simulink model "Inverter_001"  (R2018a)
settings: Solver=FixedStepDiscrete  StartTime=0.0  StopTime=inf  RelTol=1e-3  EnableMultiTasking=on
PreLoadFcn:
  | Sample_Time
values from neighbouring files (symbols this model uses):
  C_filt = 9.2e-6    (= 9.2e-06)    [master5.m]    (also in Sample_Time.m = 1.175e-06)
  Kcp = 5 /2    (= 2.5)    [master5.m]    (also in Parametri_final.m = Kcp_rac*20; Sample_Time.m = 8.8)
  Kcp0 = 5 /2    (= 2.5)    [master5.m]    (also in Parametri_final.m = Kc0p_rac*20; Sample_Time.m = 8.8)
  Kvp = 1    [master5.m]    (also in Parametri_final.m = 0.06652; Sample_Time.m = 2.4)
  Kvp0 = 1    [master5.m]    (also in Parametri_final.m = 0.06652; Sample_Time.m = 2.4)
  L_filt = 1e-3    (= 0.001)    [master5.m]    (also in Sample_Time.m = 0.01)
  Tcontrol = 5e-5     *2    (= 0.0001)    [Sample_Time.m]
  Tmeasure = 5e-5    (= 5e-05)    [Sample_Time.m]
  w = 2*pi*50    (= 314.159265359)    [master5.m]    (also in Parametri_final.m = 314.1592)
undefined symbols (not defined in the file or in its folder): A, ADCIN0, ADCIN1, ADCINA0, ADCINB0, bit, C_filtEST, CC_Tci, CC_Tci0, CC_Tcr, Compare, Control, conversion, DCAEVT1, DCAEVT1FILT, Digital, Down, ended, Event, Filtered, GPTRIP1SEL, GPTRIP2SEL, input, Module, of, Single, start, Trip, TZ1, TZ2, Up, VC_Tci, VC_Tci0, VC_Tcr, version, Zone
libraries: tiiqmathlib x92, etargetslib x20, c2802xlib x13, c2837xDlib x7, c28xdmclib x1
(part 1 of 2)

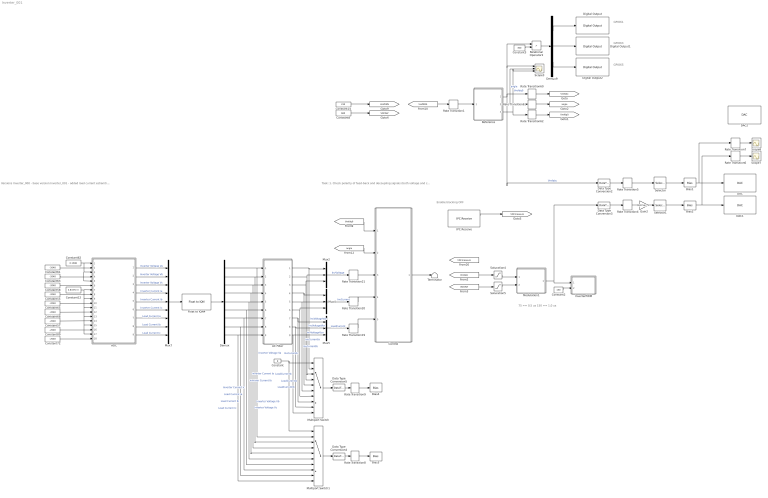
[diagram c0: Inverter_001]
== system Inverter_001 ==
  note: Enable blocking OFF
  note: Versions Inverter_000 - base version Inverter_001 - added load current estiamtion in control block
  note: Task: 1. Check polarity of feed-back and decoupling signals (both voltage and current control)
  note: 75 == 0,5 us 150 == 1,0 us
  note: GPIO61
  note: GPIO63
  note: GPIO65
  AC Filter : Subsystem
  ADC : Subsystem
  Bias1 : Bias  Bias=400
  Bias2 : Bias  Bias=400
  Bias3 : Bias  Commented=on  Bias=400
  Bias4 : Bias  Commented=on  Bias=400
  Constant : Constant  Commented=on  Value=9
  Constant12 : Constant  Value=4.8337e-3  OutDataTypeStr=single  SampleTime=0.1
  Constant14 : Constant  Value=230  OutDataTypeStr=single  SampleTime=Tcontrol
  Constant2 : Constant  Value=150  OutDataTypeStr=single
  Constant3 : Constant  Value=300  OutDataTypeStr=fixdt(1,32,2^-10,0)
  Constant{55,57..58,61,63,65,68,72,89} (9 alike) : Constant  Value=-2048  OutDataTypeStr=single  SampleTime=0.1
  Constant62 : Constant  Value=0.1588  OutDataTypeStr=single  SampleTime=0.1
  Constant8 : Constant  Value=680  OutDataTypeStr=fixdt(1,32,2^-10,0)
  Control : Subsystem
  DAC : c2837xDlib/DAC  channel=A  saturate=off
  DAC1 : c2837xDlib/DAC  channel=B  saturate=off
  DAC2 : c2837xDlib/DAC  channel=C  saturate=off
  Data Type Conversion2 : DataTypeConversion  OutDataTypeStr=single
  Data Type Conversion3 : DataTypeConversion  OutDataTypeStr=single
  Data Type Conversion4 : DataTypeConversion  Commented=on  OutDataTypeStr=single
  Data Type Conversion5 : DataTypeConversion  Commented=on  OutDataTypeStr=single
  Demux : Demux  Outputs=9
  Demux9 : Demux  Outputs=3
  Digital Output : c2837xDlib/Digital Output  GPIO_Number=GPIO56~GPIO63  GPIO_Bit0=off  GPIO_BIT0_Toggle=off  GPIO_Bit1=off  GPIO_BIT1_Toggle=off  GPIO_Bit2=off  GPIO_BIT2_Toggle=off  GPIO_Bit3=off  GPIO_BIT3_Toggle=off  GPIO_Bit4=off  GPIO_BIT4_Toggle=off  GPIO_Bit5=on  GPIO_BIT5_Toggle=off  GPIO_Bit6=off  GPIO_BIT6_Toggle=off  GPIO_Bit7=off  GPIO_BIT7_Toggle=off
  Digital Output1 : c2837xDlib/Digital Output  GPIO_Number=GPIO56~GPIO63  GPIO_Bit0=off  GPIO_BIT0_Toggle=off  GPIO_Bit1=off  GPIO_BIT1_Toggle=off  GPIO_Bit2=off  GPIO_BIT2_Toggle=off  GPIO_Bit3=off  GPIO_BIT3_Toggle=off  GPIO_Bit4=off  GPIO_BIT4_Toggle=off  GPIO_Bit5=off  GPIO_BIT5_Toggle=off  GPIO_Bit6=off  GPIO_BIT6_Toggle=off  GPIO_Bit7=on  GPIO_BIT7_Toggle=off
  Digital Output2 : c2837xDlib/Digital Output  GPIO_Number=GPIO64~GPIO71  GPIO_Bit0=off  GPIO_BIT0_Toggle=off  GPIO_Bit1=off  GPIO_BIT1_Toggle=off  GPIO_Bit2=on  GPIO_BIT2_Toggle=off  GPIO_Bit3=off  GPIO_BIT3_Toggle=off  GPIO_Bit4=off  GPIO_BIT4_Toggle=off  GPIO_Bit5=off  GPIO_BIT5_Toggle=off  GPIO_Bit6=off  GPIO_BIT6_Toggle=off  GPIO_Bit7=off  GPIO_BIT7_Toggle=off
  Float to IQN4 : tiiqmathlib/Float to IQN  Q_value=10
  Gain2 : Gain  Gain=230*sqrt(2)
  IPC Receive : c2837xDlib/IPC Receive  SelectChannel=0  DataType=single  DataLength=1  EnableBlocking=off  SampleTime=Tcontrol
  InverterPWM : Subsystem
  Modulation1 : Subsystem
  Multiport Switch : MultiPortSwitch  Commented=on  Inputs=9
  Multiport Switch1 : MultiPortSwitch  Commented=on  Inputs=9
  Mux2 : Mux  Inputs=3
  Mux4 : Mux  Inputs=3
  Mux5 : Mux  Inputs=3
  Mux7 : Mux  Inputs=9
  Rate Transition1 : RateTransition  OutPortSampleTime=5e-5
  Rate Transition{4..5,19..21,60..62} (8 alike) : RateTransition  OutPortSampleTime=Tcontrol
  Rate Transition6 : RateTransition  OutPortSampleTime=2e-4
  Rate Transition7 : RateTransition  OutPortSampleTime=2e-4
  Rate Transition8 : RateTransition  Commented=on  OutPortSampleTime=Tcontrol
  Rate Transition9 : RateTransition  Commented=on  OutPortSampleTime=Tcontrol
  Reference : Subsystem
  Relational Operator2 : RelationalOperator  Operator=>  OutDataTypeStr=boolean
  Saturation4 : Saturate  UpperLimit=400  LowerLimit=-400
  Saturation5 : Saturate  UpperLimit=720  LowerLimit=0
  Scope3 : Scope  NumInputPorts=3
  Scope7 : Scope
  Scope8 : Scope
  Selector : Selector  InputPortWidth=3  IndexOptions=Index vector (dialog)  Indices=[2]  OutputSizes=1
  Selector1 : Selector  InputPortWidth=4  IndexOptions=Index vector (dialog)  Indices=[2]  OutputSizes=1
  Terminator : Terminator
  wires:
  Constant8/1 -> [VDCRef]
  [Vrefabc] -> Saturation4/1
  [angle] -> Control/2(Angle)
  Constant2/1 -> InverterPWM/2(DeadBand)
  Float to IQN4/1 -> Demux/1
  Constant68/1 -> ADC/12(" ADC-A4 Offset")
  Saturation4/1 -> Modulation1/1(Vcontrol)
  Modulation1/1(VPWM) -> Data Type Conversion3/1, InverterPWM/1(PWM)
  Saturation5/1 -> Modulation1/2(VDC)
  AC Filter/1(Out1) -> Multiport Switch/2, Mux2/1  "InvVoltageVan"
  Rate Transition21/1 -> Control/3(Vabc Phase)
  Mux2/1 -> Rate Transition21/1  "InvVoltage"
  [Vrefdq0] -> Control/1(dq0Ref)
  [VDCRef] -> Saturation5/1
  Constant89/1 -> ADC/16(" ADC-C3 Offset")
  AC Filter/4(Out4) -> Multiport Switch/5, Mux4/1  "InvCurrentIa"
  Control/1(Vabc Control) -> Terminator/1
  Rate Transition20/1 -> Control/4(Iabc Inv)
  AC Filter/6(Out6) -> Multiport Switch/7, Mux4/3  "InvCurrentIc"
  AC Filter/9(Out9) -> Mux5/3, Multiport Switch/10  "LoadCurrentIc"
  Mux5/1 -> Rate Transition19/1  "LoadCurrent"
  AC Filter/8(Out8) -> Multiport Switch/9, Mux5/2  "LoadCurrentIb"
  AC Filter/3(Out3) -> Multiport Switch/4, Mux2/3  "InvVoltageVcn"
  AC Filter/5(Out5) -> Multiport Switch/6, Mux4/2  "InvCurrentIb"
  AC Filter/7(Out7) -> Multiport Switch/8, Mux5/1  "LoadCurentIa"
  Constant65/1 -> ADC/10(" ADC-A3 Offset")
  Constant62/1 -> ADC/5(ADC-D4 Scaling), ADC/3(ADC-D3 Scaling), ADC/1(ADC-D2 Scaling)
  Rate Transition19/1 -> Control/5(Iabc Load)
  Constant63/1 -> ADC/4(" ADC-D3 Offset")
  Constant55/1 -> ADC/8(" ADC-A2 Offset")
  Constant61/1 -> ADC/2(" ADC-D2 Offset")
  Constant14/1 -> [VrefRMS]
  Mux7/1 -> Float to IQN4/1
  Constant12/1 -> ADC/9(ADC-A3 Scaling), ADC/11(ADC-A4 Scaling), ADC/13(ADC-C2 Scaling), ADC/15(" ADC-C3 Scaling"), ADC/17(ADC-C4 Scaling), ADC/7(ADC-A2 Scaling)
  Constant72/1 -> ADC/18(" ADC-C4 Offset")
  Constant57/1 -> ADC/14(" ADC-C2 Offset")
  AC Filter/2(Out2) -> Multiport Switch/3, Mux2/2  "InvVoltageVbn"
  Constant58/1 -> ADC/6(" ADC-D4 Offset")
  Mux4/1 -> Rate Transition20/1  "InvCurrent"
  Demux9/2 -> Digital Output1/1
  Rate Transition1/1 -> Reference/1(Vac Ref)
  [VrefRMS] -> Rate Transition1/1
  Rate Transition61/1 -> [angle]
  Reference/3(dq0) -> Scope3/3, Rate Transition62/1  "Vrefdq0"
  Rate Transition62/1 -> [Vrefdq0]
  Reference/1(abc) -> Data Type Conversion2/1, Scope3/1, Relational Operator2/1, Rate Transition60/1  "Vrefabc"
  Demux9/3 -> Digital Output2/1
  Reference/2(angle) -> Scope3/2, Rate Transition61/1  "angle"
  Rate Transition60/1 -> [Vrefabc]
  Demux9/1 -> Digital Output/1
  Relational Operator2/1 -> Demux9/1
  Constant3/1 -> Relational Operator2/2
  ADC/1(ADC-D2) -> Mux7/1  "Inverter Voltage Va"
  ADC/2(ADC-D3) -> Mux7/2  "Inverter Voltage Vb"
  ADC/3(ADC-D4) -> Mux7/3  "Inverter Voltage Vc"
  ADC/4(ADC-A2) -> Mux7/4  "Inverter Current Ia"
  ADC/5(ADC-A3) -> Mux7/5  "Inverter Current Ib"
  ADC/6(ADC-A4) -> Mux7/6  "Inverter Current Ic"
  ADC/7(ADC-C2) -> Mux7/7  "Load Current Ia"
  ADC/8(ADC-C3) -> Mux7/8  "Load Current Ib"
  ADC/9(ADC-C4) -> Mux7/9  "Load Current Ic"
  Demux/1 -> Multiport Switch1/2, AC Filter/1(In1)  "Inverter Voltage Va"
  Demux/2 -> Multiport Switch1/3, AC Filter/2(In2)  "Inverter Voltage Vb"
  Demux/3 -> Multiport Switch1/4, AC Filter/3(In3)  "Inverter Voltage Vc"
  Demux/4 -> Multiport Switch1/5, AC Filter/4(In4)  "Inverter Current Ia"
  Demux/5 -> Multiport Switch1/6, AC Filter/5(In5)  "Inverter Current Ib"
  Demux/6 -> Multiport Switch1/7, AC Filter/6(In6)  "Inverter Current Ic"
  Demux/7 -> Multiport Switch1/8, AC Filter/7(In7)  "Load Current Ia"
  Demux/8 -> Multiport Switch1/9, AC Filter/8(In8)  "Load Current Ib"
  Demux/9 -> Multiport Switch1/10, AC Filter/9(In9)  "Load Current Ic"
  Rate Transition4/1 -> Gain2/1
  Rate Transition5/1 -> Selector/1
  Data Type Conversion2/1 -> Rate Transition5/1
  Data Type Conversion3/1 -> Rate Transition4/1
  Gain2/1 -> Selector1/1
  Selector/1 -> Bias1/1
  Selector1/1 -> Bias2/1
  Bias1/1 -> Rate Transition7/1, DAC/1
  Bias2/1 -> DAC1/1, Rate Transition6/1
  Rate Transition6/1 -> Scope7/1
  Rate Transition7/1 -> Scope8/1
  Data Type Conversion4/1 -> Rate Transition8/1
  Rate Transition8/1 -> Bias3/1
  Rate Transition9/1 -> Bias4/1
  Data Type Conversion5/1 -> Rate Transition9/1
  Constant/1 -> Multiport Switch1/1, Multiport Switch/1
  Multiport Switch/1 -> Data Type Conversion5/1
  Multiport Switch1/1 -> Data Type Conversion4/1
  IPC Receive/1 -> [VDCmeasure]

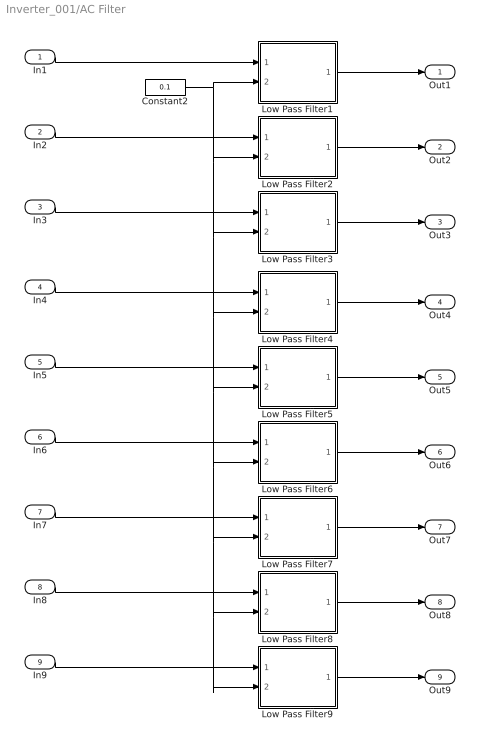
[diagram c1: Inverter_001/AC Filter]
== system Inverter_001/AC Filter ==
  In1 : Inport
  In2 : Inport  Port=2
  In3 : Inport  Port=3
  In4 : Inport  Port=4
  In5 : Inport  Port=5
  In6 : Inport  Port=6
  In7 : Inport  Port=7
  In8 : Inport  Port=8
  In9 : Inport  Port=9
  Constant2 : Constant  Value=0.1  OutDataTypeStr=fixdt(1,32,2^-10,0)
  Low Pass Filter1 : Subsystem  AncestorBlock=LCPMeasure/High Pass Filter
      mask help: <!DOCTYPE HTML PUBLIC "-//W3C//DTD HTML 4.01 Transitional//EN"> <html><head> </head> <body> <p style="text-align: center; font-weight: bold;">High Pass Filter </p> <p><strong>Inputs: </strong></p> <ol> <li>Input (single)</li> <li>Sample Time (single)</li> <li>Time Constant (single)</li> </ol> <p><strong>Outputs: </strong></p> <ol> <li>Output (single)</li> </ol> </body></html>
  Low Pass Filter2 : Subsystem  AncestorBlock=LCPMeasure/High Pass Filter
      mask help: <!DOCTYPE HTML PUBLIC "-//W3C//DTD HTML 4.01 Transitional//EN"> <html><head> </head> <body> <p style="text-align: center; font-weight: bold;">High Pass Filter </p> <p><strong>Inputs: </strong></p> <ol> <li>Input (single)</li> <li>Sample Time (single)</li> <li>Time Constant (single)</li> </ol> <p><strong>Outputs: </strong></p> <ol> <li>Output (single)</li> </ol> </body></html>
  Low Pass Filter3 : Subsystem  AncestorBlock=LCPMeasure/High Pass Filter
      mask help: <!DOCTYPE HTML PUBLIC "-//W3C//DTD HTML 4.01 Transitional//EN"> <html><head> </head> <body> <p style="text-align: center; font-weight: bold;">High Pass Filter </p> <p><strong>Inputs: </strong></p> <ol> <li>Input (single)</li> <li>Sample Time (single)</li> <li>Time Constant (single)</li> </ol> <p><strong>Outputs: </strong></p> <ol> <li>Output (single)</li> </ol> </body></html>
  Low Pass Filter4 : Subsystem  AncestorBlock=LCPMeasure/High Pass Filter
      mask help: <!DOCTYPE HTML PUBLIC "-//W3C//DTD HTML 4.01 Transitional//EN"> <html><head> </head> <body> <p style="text-align: center; font-weight: bold;">High Pass Filter </p> <p><strong>Inputs: </strong></p> <ol> <li>Input (single)</li> <li>Sample Time (single)</li> <li>Time Constant (single)</li> </ol> <p><strong>Outputs: </strong></p> <ol> <li>Output (single)</li> </ol> </body></html>
  Low Pass Filter5 : Subsystem  AncestorBlock=LCPMeasure/High Pass Filter
      mask help: <!DOCTYPE HTML PUBLIC "-//W3C//DTD HTML 4.01 Transitional//EN"> <html><head> </head> <body> <p style="text-align: center; font-weight: bold;">High Pass Filter </p> <p><strong>Inputs: </strong></p> <ol> <li>Input (single)</li> <li>Sample Time (single)</li> <li>Time Constant (single)</li> </ol> <p><strong>Outputs: </strong></p> <ol> <li>Output (single)</li> </ol> </body></html>
  Low Pass Filter6 : Subsystem  AncestorBlock=LCPMeasure/High Pass Filter
      mask help: <!DOCTYPE HTML PUBLIC "-//W3C//DTD HTML 4.01 Transitional//EN"> <html><head> </head> <body> <p style="text-align: center; font-weight: bold;">High Pass Filter </p> <p><strong>Inputs: </strong></p> <ol> <li>Input (single)</li> <li>Sample Time (single)</li> <li>Time Constant (single)</li> </ol> <p><strong>Outputs: </strong></p> <ol> <li>Output (single)</li> </ol> </body></html>
  Low Pass Filter7 : Subsystem  AncestorBlock=LCPMeasure/High Pass Filter
      mask help: <!DOCTYPE HTML PUBLIC "-//W3C//DTD HTML 4.01 Transitional//EN"> <html><head> </head> <body> <p style="text-align: center; font-weight: bold;">High Pass Filter </p> <p><strong>Inputs: </strong></p> <ol> <li>Input (single)</li> <li>Sample Time (single)</li> <li>Time Constant (single)</li> </ol> <p><strong>Outputs: </strong></p> <ol> <li>Output (single)</li> </ol> </body></html>
  Low Pass Filter8 : Subsystem  AncestorBlock=LCPMeasure/High Pass Filter
      mask help: <!DOCTYPE HTML PUBLIC "-//W3C//DTD HTML 4.01 Transitional//EN"> <html><head> </head> <body> <p style="text-align: center; font-weight: bold;">High Pass Filter </p> <p><strong>Inputs: </strong></p> <ol> <li>Input (single)</li> <li>Sample Time (single)</li> <li>Time Constant (single)</li> </ol> <p><strong>Outputs: </strong></p> <ol> <li>Output (single)</li> </ol> </body></html>
  Low Pass Filter9 : Subsystem  AncestorBlock=LCPMeasure/High Pass Filter
      mask help: <!DOCTYPE HTML PUBLIC "-//W3C//DTD HTML 4.01 Transitional//EN"> <html><head> </head> <body> <p style="text-align: center; font-weight: bold;">High Pass Filter </p> <p><strong>Inputs: </strong></p> <ol> <li>Input (single)</li> <li>Sample Time (single)</li> <li>Time Constant (single)</li> </ol> <p><strong>Outputs: </strong></p> <ol> <li>Output (single)</li> </ol> </body></html>
  Out1 : Outport
  Out2 : Outport  Port=2
  Out3 : Outport  Port=3
  Out4 : Outport  Port=4
  Out5 : Outport  Port=5
  Out6 : Outport  Port=6
  Out7 : Outport  Port=7
  Out8 : Outport  Port=8
  Out9 : Outport  Port=9
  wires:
  Constant2/1 -> Low Pass Filter2/2(TimeConstant), Low Pass Filter3/2(TimeConstant), Low Pass Filter4/2(TimeConstant), Low Pass Filter5/2(TimeConstant), Low Pass Filter6/2(TimeConstant), Low Pass Filter7/2(TimeConstant), Low Pass Filter9/2(TimeConstant), Low Pass Filter8/2(TimeConstant), Low Pass Filter1/2(TimeConstant)
  In9/1 -> Low Pass Filter9/1(Input)
  In2/1 -> Low Pass Filter2/1(Input)
  In7/1 -> Low Pass Filter7/1(Input)
  In3/1 -> Low Pass Filter3/1(Input)
  In4/1 -> Low Pass Filter4/1(Input)
  In5/1 -> Low Pass Filter5/1(Input)
  In6/1 -> Low Pass Filter6/1(Input)
  In8/1 -> Low Pass Filter8/1(Input)
  Low Pass Filter3/1(Output) -> Out3/1
  Low Pass Filter4/1(Output) -> Out4/1
  Low Pass Filter5/1(Output) -> Out5/1
  Low Pass Filter2/1(Output) -> Out2/1
  Low Pass Filter6/1(Output) -> Out6/1
  Low Pass Filter8/1(Output) -> Out8/1
  Low Pass Filter1/1(Output) -> Out1/1
  Low Pass Filter9/1(Output) -> Out9/1
  Low Pass Filter7/1(Output) -> Out7/1
  In1/1 -> Low Pass Filter1/1(Input)

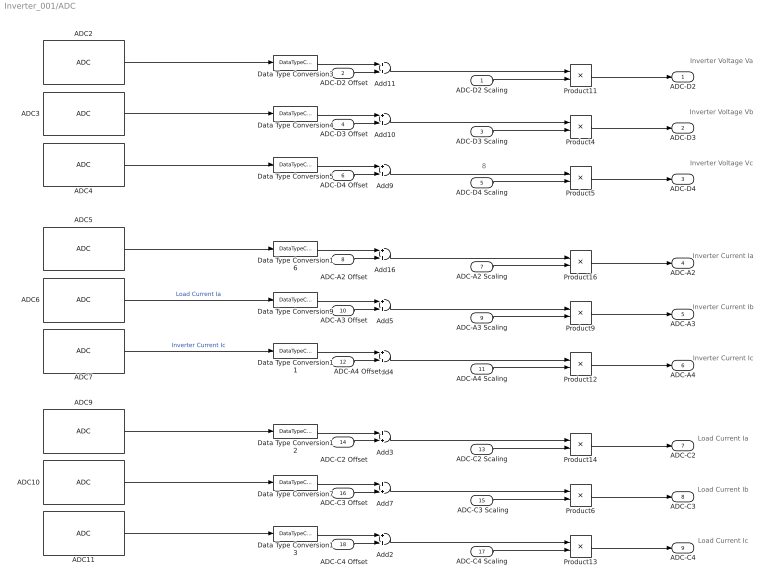
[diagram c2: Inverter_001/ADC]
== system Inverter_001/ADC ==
  note: Inverter Voltage Va
  note: Inverter Current Ia
  note: 8
  note: Inverter Current Ib
  note: Inverter Current Ic
  note: Load Current Ia
  note: Load Current Ib
  note: Load Current Ic
  note: Inverter Voltage Vb
  note: Inverter Voltage Vc
  ADC-D2 Scaling : Inport
  " ADC-D2 Offset" : Inport  Port=2
  ADC-D3 Scaling : Inport  Port=3
  " ADC-D3 Offset" : Inport  Port=4
  ADC-D4 Scaling : Inport  Port=5
  " ADC-D4 Offset" : Inport  Port=6
  ADC-A2 Scaling : Inport  Port=7
  " ADC-A2 Offset" : Inport  Port=8
  ADC-A3 Scaling : Inport  Port=9
  " ADC-A3 Offset" : Inport  Port=10
  ADC-A4 Scaling : Inport  Port=11
  " ADC-A4 Offset" : Inport  Port=12
  ADC-C2 Scaling : Inport  Port=13
  " ADC-C2 Offset" : Inport  Port=14
  " ADC-C3 Scaling" : Inport  Port=15
  " ADC-C3 Offset" : Inport  Port=16
  ADC-C4 Scaling : Inport  Port=17
  " ADC-C4 Offset" : Inport  Port=18
  ADC10 : c2802xlib/ADC  blkParamProc=C2000_Type4  ADCModule=C  samplingMode=Single sample mode  ADCResolution=12-bit (Single-ended input)  useSOC1=SOC11  useSOC2=SOC0_SOC1  SOCAcquisitionWindow=15  SOCTriggerSource=Software  SOCInterruptTrigger=ADCINT1  Ts=Tmeasure  dType=uint16  postInterrupt=off  interruptSel=ADCINT1  ADCINTContinuous=on  endma=off  chdma=1  conv1=ADCINA0  conv2=ADCINA0 and ADCINB0  conv1_Type4=ADCIN3  conv2_Type4=ADCIN0 and ADCIN1
  ADC11 : c2802xlib/ADC  blkParamProc=C2000_Type4  ADCModule=C  samplingMode=Single sample mode  ADCResolution=12-bit (Single-ended input)  useSOC1=SOC12  useSOC2=SOC0_SOC1  SOCAcquisitionWindow=15  SOCTriggerSource=Software  SOCInterruptTrigger=ADCINT1  Ts=Tmeasure  dType=uint16  postInterrupt=off  interruptSel=ADCINT1  ADCINTContinuous=on  endma=off  chdma=1  conv1=ADCINA0  conv2=ADCINA0 and ADCINB0  conv1_Type4=ADCIN4  conv2_Type4=ADCIN0 and ADCIN1
  ADC2 : c2802xlib/ADC  blkParamProc=C2000_Type4  ADCModule=D  samplingMode=Single sample mode  ADCResolution=12-bit (Single-ended input)  useSOC1=SOC2  useSOC2=SOC0_SOC1  SOCAcquisitionWindow=15  SOCTriggerSource=Software  SOCInterruptTrigger=ADCINT1  Ts=Tmeasure  dType=uint16  postInterrupt=off  interruptSel=ADCINT1  ADCINTContinuous=on  endma=off  chdma=1  conv1=ADCINA0  conv2=ADCINA0 and ADCINB0  conv1_Type4=ADCIN2  conv2_Type4=ADCIN0 and ADCIN1
  ADC3 : c2802xlib/ADC  blkParamProc=C2000_Type4  ADCModule=D  samplingMode=Single sample mode  ADCResolution=12-bit (Single-ended input)  useSOC1=SOC5  useSOC2=SOC0_SOC1  SOCAcquisitionWindow=15  SOCTriggerSource=Software  SOCInterruptTrigger=ADCINT1  Ts=Tmeasure  dType=uint16  postInterrupt=off  interruptSel=ADCINT1  ADCINTContinuous=on  endma=off  chdma=1  conv1=ADCINA0  conv2=ADCINA0 and ADCINB0  conv1_Type4=ADCIN3  conv2_Type4=ADCIN0 and ADCIN1
  ADC4 : c2802xlib/ADC  blkParamProc=C2000_Type4  ADCModule=D  samplingMode=Single sample mode  ADCResolution=12-bit (Single-ended input)  useSOC1=SOC7  useSOC2=SOC0_SOC1  SOCAcquisitionWindow=15  SOCTriggerSource=Software  SOCInterruptTrigger=ADCINT1  Ts=Tmeasure  dType=uint16  postInterrupt=off  interruptSel=ADCINT1  ADCINTContinuous=on  endma=off  chdma=1  conv1=ADCINA0  conv2=ADCINA0 and ADCINB0  conv1_Type4=ADCIN4  conv2_Type4=ADCIN0 and ADCIN1
  ADC5 : c2802xlib/ADC  blkParamProc=C2000_Type4  ADCModule=A  samplingMode=Single sample mode  ADCResolution=12-bit (Single-ended input)  useSOC1=SOC4  useSOC2=SOC0_SOC1  SOCAcquisitionWindow=15  SOCTriggerSource=Software  SOCInterruptTrigger=ADCINT1  Ts=Tmeasure  dType=uint16  postInterrupt=off  interruptSel=ADCINT1  ADCINTContinuous=on  endma=off  chdma=1  conv1=ADCINA0  conv2=ADCINA0 and ADCINB0  conv1_Type4=ADCIN2  conv2_Type4=ADCIN0 and ADCIN1
  ADC6 : c2802xlib/ADC  blkParamProc=C2000_Type4  ADCModule=A  samplingMode=Single sample mode  ADCResolution=12-bit (Single-ended input)  useSOC1=SOC6  useSOC2=SOC0_SOC1  SOCAcquisitionWindow=15  SOCTriggerSource=Software  SOCInterruptTrigger=ADCINT1  Ts=Tmeasure  dType=uint16  postInterrupt=off  interruptSel=ADCINT1  ADCINTContinuous=on  endma=off  chdma=1  conv1=ADCINA0  conv2=ADCINA0 and ADCINB0  conv1_Type4=ADCIN3  conv2_Type4=ADCIN0 and ADCIN1
  ADC7 : c2802xlib/ADC  blkParamProc=C2000_Type4  ADCModule=A  samplingMode=Single sample mode  ADCResolution=12-bit (Single-ended input)  useSOC1=SOC8  useSOC2=SOC0_SOC1  SOCAcquisitionWindow=15  SOCTriggerSource=Software  SOCInterruptTrigger=ADCINT1  Ts=Tmeasure  dType=uint16  postInterrupt=off  interruptSel=ADCINT1  ADCINTContinuous=on  endma=off  chdma=1  conv1=ADCINA0  conv2=ADCINA0 and ADCINB0  conv1_Type4=ADCIN4  conv2_Type4=ADCIN0 and ADCIN1
  ADC9 : c2802xlib/ADC  blkParamProc=C2000_Type4  ADCModule=C  samplingMode=Single sample mode  ADCResolution=12-bit (Single-ended input)  useSOC1=SOC10  useSOC2=SOC0_SOC1  SOCAcquisitionWindow=15  SOCTriggerSource=Software  SOCInterruptTrigger=ADCINT1  Ts=Tmeasure  dType=uint16  postInterrupt=off  interruptSel=ADCINT1  ADCINTContinuous=on  endma=off  chdma=1  conv1=ADCINA0  conv2=ADCINA0 and ADCINB0  conv1_Type4=ADCIN2  conv2_Type4=ADCIN0 and ADCIN1
  Add{2..5,7,9..11,16} (9 alike) : Sum
  Data Type Conversion{3..5,7,9,11..13,16} (9 alike) : DataTypeConversion  OutDataTypeStr=single
  Product{4..6,9,11..14,16} (9 alike) : Product
  ADC-D2 : Outport
  ADC-D3 : Outport  Port=2
  ADC-D4 : Outport  Port=3
  ADC-A2 : Outport  Port=4
  ADC-A3 : Outport  Port=5
  ADC-A4 : Outport  Port=6
  ADC-C2 : Outport  Port=7
  ADC-C3 : Outport  Port=8
  ADC-C4 : Outport  Port=9
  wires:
  Data Type Conversion11/1 -> Add4/1
  Product5/1 -> ADC-D4/1
  Data Type Conversion5/1 -> Add9/1
  ADC4/1 -> Data Type Conversion5/1
  Product11/1 -> ADC-D2/1
  ADC2/1 -> Data Type Conversion3/1
  Product13/1 -> ADC-C4/1
  Data Type Conversion9/1 -> Add5/1
  ADC7/1 -> Data Type Conversion11/1  "Inverter Current Ic"
  ADC3/1 -> Data Type Conversion4/1
  Product6/1 -> ADC-C3/1
  ADC-D4 Scaling/1 -> Product5/2
  Product12/1 -> ADC-A4/1
  Add11/1 -> Product11/1
  Data Type Conversion12/1 -> Add3/1
  Product14/1 -> ADC-C2/1
  ADC-C4 Scaling/1 -> Product13/2
  Add2/1 -> Product13/1
  Add5/1 -> Product9/1
  Add7/1 -> Product6/1
  Data Type Conversion7/1 -> Add7/1
  ADC-C2 Scaling/1 -> Product14/2
  Data Type Conversion4/1 -> Add10/1
  Data Type Conversion13/1 -> Add2/1
  Add3/1 -> Product14/1
  ADC10/1 -> Data Type Conversion7/1
  Add4/1 -> Product12/1
  Data Type Conversion3/1 -> Add11/1
  Product4/1 -> ADC-D3/1
  ADC6/1 -> Data Type Conversion9/1  "Load Current Ia"
  ADC11/1 -> Data Type Conversion13/1
  Product9/1 -> ADC-A3/1
  ADC9/1 -> Data Type Conversion12/1
  Add10/1 -> Product4/1
  Add9/1 -> Product5/1
  ADC-D2 Scaling/1 -> Product11/2
  ADC-A3 Scaling/1 -> Product9/2
  ADC-A4 Scaling/1 -> Product12/2
  " ADC-C3 Scaling"/1 -> Product6/2
  ADC-D3 Scaling/1 -> Product4/2
  " ADC-C3 Offset"/1 -> Add7/2
  " ADC-D4 Offset"/1 -> Add9/2
  " ADC-C4 Offset"/1 -> Add2/2
  " ADC-C2 Offset"/1 -> Add3/2
  " ADC-A4 Offset"/1 -> Add4/2
  " ADC-A3 Offset"/1 -> Add5/2
  " ADC-D3 Offset"/1 -> Add10/2
  " ADC-D2 Offset"/1 -> Add11/2
  Product16/1 -> ADC-A2/1
  Add16/1 -> Product16/1
  Data Type Conversion16/1 -> Add16/1
  ADC-A2 Scaling/1 -> Product16/2
  " ADC-A2 Offset"/1 -> Add16/2
  ADC5/1 -> Data Type Conversion16/1

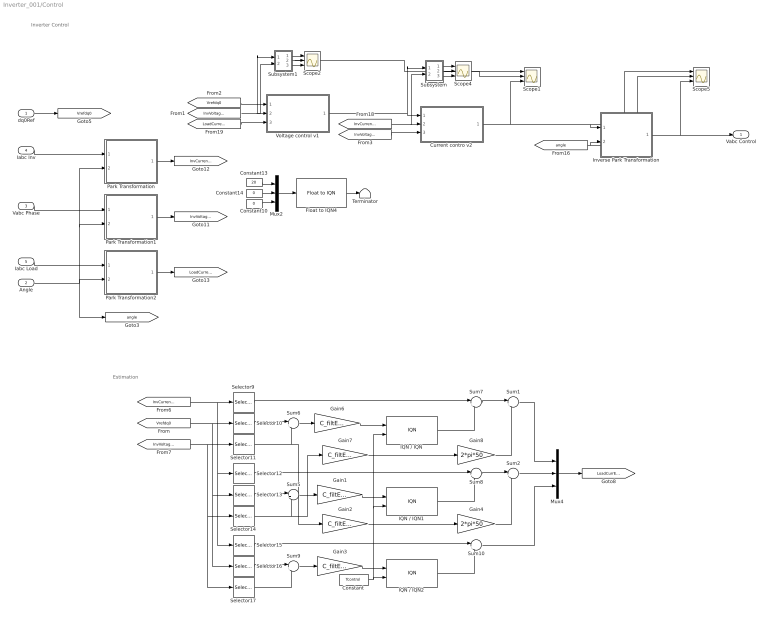
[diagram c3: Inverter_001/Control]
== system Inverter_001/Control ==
  note: Estimation
  note: Inverter Control
  dq0Ref : Inport
  Angle : Inport  Port=2
  Vabc Phase : Inport  Port=3
  Iabc Inv : Inport  Port=4
  Iabc Load : Inport  Port=5
  Constant : Constant  Commented=on  Value=Tcontrol
  Constant10 : Constant  Value=0  OutDataTypeStr=single
  Constant13 : Constant  Value=20  OutDataTypeStr=single
  Constant14 : Constant  Value=0  OutDataTypeStr=single
  Current contro v2 : Subsystem
  Float to IQN4 : tiiqmathlib/Float to IQN  Q_value=10
  Gain{1..3,6..7} (5 alike) : Gain  Commented=on  Gain=C_filtEST
  Gain4 : Gain  Commented=on  Gain=2*pi*50
  Gain8 : Gain  Commented=on  Gain=2*pi*50
  IQN / IQN : tiiqmathlib/IQN // IQN  Commented=on
  IQN / IQN1 : tiiqmathlib/IQN // IQN  Commented=on
  IQN / IQN2 : tiiqmathlib/IQN // IQN  Commented=on
  Inverse Park Transformation : Subsystem  InitFcn=tic2000lib_licenseCheck  mask(Inverse Park Transformation){}
      mask help: This block performs vector transformation from orthogonal rotating reference frame into orthogonal stationary frame. All inputs and outputs are signed 32-bit fixed-point numbers with Q value between 1 and 29.
  Mux2 : Mux  Inputs=3
  Mux4 : Mux  Commented=on  Inputs=3
  Park Transformation : Subsystem  InitFcn=tic2000lib_licenseCheck  mask(Inverse Park Transformation){}
      mask help: This block performs vector transformation from orthogonal rotating reference frame into orthogonal stationary frame. All inputs and outputs are signed 32-bit fixed-point numbers with Q value between 1 and 29.
  Park Transformation1 : Subsystem  InitFcn=tic2000lib_licenseCheck  mask(Inverse Park Transformation){}
      mask help: This block performs vector transformation from orthogonal rotating reference frame into orthogonal stationary frame. All inputs and outputs are signed 32-bit fixed-point numbers with Q value between 1 and 29.
  Park Transformation2 : Subsystem  InitFcn=tic2000lib_licenseCheck  mask(Inverse Park Transformation){}
      mask help: This block performs vector transformation from orthogonal rotating reference frame into orthogonal stationary frame. All inputs and outputs are signed 32-bit fixed-point numbers with Q value between 1 and 29.
  Scope{1..2,4..5} (4 alike) : Scope  NumInputPorts=3
  Selector10 : Selector  Commented=on  InputPortWidth=3  IndexOptions=Index vector (dialog)  Indices=[1]  OutputSizes=1
  Selector11 : Selector  Commented=on  InputPortWidth=3  IndexOptions=Index vector (dialog)  Indices=[1]  OutputSizes=1
  Selector12 : Selector  Commented=on  InputPortWidth=3  IndexOptions=Index vector (dialog)  Indices=[2]  OutputSizes=1
  Selector13 : Selector  Commented=on  InputPortWidth=3  IndexOptions=Index vector (dialog)  Indices=[2]  OutputSizes=1
  Selector14 : Selector  Commented=on  InputPortWidth=3  IndexOptions=Index vector (dialog)  Indices=[2]  OutputSizes=1
  Selector15 : Selector  Commented=on  InputPortWidth=3  IndexOptions=Index vector (dialog)  Indices=[3]  OutputSizes=1
  Selector16 : Selector  Commented=on  InputPortWidth=3  IndexOptions=Index vector (dialog)  Indices=[3]  OutputSizes=1
  Selector17 : Selector  Commented=on  InputPortWidth=3  IndexOptions=Index vector (dialog)  Indices=[3]  OutputSizes=1
  Selector9 : Selector  Commented=on  InputPortWidth=3  IndexOptions=Index vector (dialog)  Indices=[1]  OutputSizes=1
  Subsystem : Subsystem  Commented=on
  Subsystem1 : Subsystem  Commented=on
  Sum1 : Sum  Commented=on  Inputs=|++
  Sum{2,5..10} (7 alike) : Sum  Commented=on  Inputs=|+-
  Terminator : Terminator
  Voltage control v1 : Subsystem
  Vabc Control : Outport
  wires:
  Inverse Park Transformation/1(ABC) -> Vabc Control/1, Scope5/3
  Float to IQN4/1 -> Terminator/1
  [LoadCurrentdq0] -> Voltage control v1/3(Id,q,0_load)
  [InvVoltagedq0] -> Current contro v2/3(Vd,q,0_load)
  Voltage control v1/1(Id,q,0_ref) -> Subsystem/1(I1), Current contro v2/1(Id,q,0_ref)
  [InvVoltagedq0] -> Subsystem1/1(I1), Subsystem1/2(I2), Voltage control v1/2(Vd,q,0_load)
  [angle] -> Scope5/2, Inverse Park Transformation/2(theta)
  Subsystem1/2(O2) -> Scope1/1, Scope2/2
  Iabc Load/1 -> Park Transformation2/1(ABC)
  Subsystem/2(O2) -> Scope1/2, Scope4/2
  Park Transformation2/1(DQ0) -> [LoadCurrentdq0]
  Park Transformation/1(DQ0) -> [InvCurrentdq0]
  Subsystem1/3(O3) -> Scope2/3
  Park Transformation1/1(DQ0) -> [InvVoltagedq0]
  Vabc Phase/1 -> Park Transformation1/1(ABC)
  Iabc Inv/1 -> Park Transformation/1(ABC)
  Mux2/1 -> Float to IQN4/1
  [InvCurrentdq0] -> Current contro v2/2(Id,q,0), Subsystem/2(I2)
  Angle/1 -> Park Transformation/2(theta), Park Transformation1/2(theta), Park Transformation2/2(theta), [angle]
  Subsystem/3(O3) -> Scope4/3
  Subsystem/1(O1) -> Scope4/1
  Subsystem1/1(O1) -> Scope2/1
  dq0Ref/1 -> [Vrefdq0]
  Constant13/1 -> Mux2/1
  Constant14/1 -> Mux2/2
  Current contro v2/1(Vd,q,0_PWM) -> Scope5/1, Inverse Park Transformation/1(DQ0), Scope1/3
  [Vrefdq0] -> Voltage control v1/1(Vd,q,0_ref)
  Constant10/1 -> Mux2/3
  Mux4/1 -> [LoadCurrEstdq0]
  Sum8/1 -> Sum2/1
  Gain8/1 -> Sum1/2
  Gain7/1 -> Gain8/1
  Gain2/1 -> Gain4/1
  Gain4/1 -> Sum2/2
  Sum7/1 -> Sum1/1
  Sum10/1 -> Mux4/3
  Sum2/1 -> Mux4/2
  Sum1/1 -> Mux4/1
  Selector17/1 -> Sum9/2
  Sum9/1 -> Gain3/1
  IQN / IQN2/1 -> Sum10/2
  Gain3/1 -> IQN / IQN2/1
  Selector15/1 -> Sum10/1
  Selector16/1 -> Sum9/1
  Selector14/1 -> Sum5/2, Gain7/1
  Sum5/1 -> Gain1/1
  IQN / IQN1/1 -> Sum8/2
  Gain1/1 -> IQN / IQN1/1
  Selector12/1 -> Sum8/1
  Selector13/1 -> Sum5/1
  [InvVoltagedq0] -> Selector14/1, Selector17/1, Selector11/1
  [Vrefdq0] -> Selector16/1, Selector13/1, Selector10/1
  [InvCurrentdq0] -> Selector12/1, Selector15/1, Selector9/1
  Selector11/1 -> Sum6/2, Gain2/1
  Sum6/1 -> Gain6/1
  IQN / IQN/1 -> Sum7/2
  Gain6/1 -> IQN / IQN/1
  Selector9/1 -> Sum7/1
  Selector10/1 -> Sum6/1
  Constant/1 -> IQN / IQN1/2, IQN / IQN/2, IQN / IQN2/2

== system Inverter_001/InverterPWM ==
  PWM : Inport
  DeadBand : Inport  Port=2
  Add{,13..15} (4 alike) : Sum
  Constant13 : Constant  Value=0.5  OutDataTypeStr=single
  Constant14 : Constant  Value=12500  OutDataTypeStr=single
  Constant15 : Constant  OutDataTypeStr=single
  Demux5 : Demux
  Product{,15..21} (8 alike) : Product
  ePWM : c2802xlib/ePWM  useModule=ePWM5  ePWMxLINKTBPRD=Not Linked  periodUnits=Clock cycles  timerSource=Specify via dialog  timerPeriod_clk=12500  timerPeriod_sec=0.0001  tbshadow=Counter equals to zero  countingMode=Up-Down  phaseActiveEnable=Disable  phaseDirection=Count down after sync  phaseActive=0  synchronizationEnable=off  dcaevt1Sync=off  dcbevt1Sync=off  synchronizationOption=Disable  clockPrescale=1  HSclockPrescale=1  enswap=off  ePWMxAStatus=on  ePWMxAactionLogic1=Set  ePWMxAactionLogic2=Clear  ePWMxAactionLogic3=Clear  ePWMxAactionLogic4=Set  ePWMxAactionLogic5=Do nothing  ePWMxAactionLogic6=Do nothing  ePWMxALoadMode=Load on counter equals to zero (CTR=Zero)  ePWMxACSFenable=off  ePWMxACSFvalue=Forcing disable  ePWMxASFreload=Zero  ePWMxBStatus=on  ePWMxBactionLogic1=Clear  ePWMxBactionLogic2=Set  ePWMxBactionLogic3=Do nothing  ePWMxBactionLogic4=Do nothing  ePWMxBactionLogic5=Set  ePWMxBactionLogic6=Clear  ePWMxBLoadMode=Load on counter equals to zero (CTR=Zero)  ePWMxBCSFenable=off  ePWMxBCSFvalue=Forcing disable  ePWMxBSFreload=Zero  ePWNxBOutWay=off  ePWMxLINKCMPA=Not Linked  CMPAUnits=Clock cycles  CMPASource=Input port  CMPAValue_per=50  CMPAValue_clk=3750  enCMPAshadow=Counter equals to zero  ePWMxLINKCMPB=Not Linked  CMPBUnits=Clock cycles  CMPBSource=Input port  CMPBValue_per=50  CMPBValue_clk=3750  enCMPBshadow=Counter equals to zero  ePWMxLINKCMPC=Not Linked  CMPCUnits=Clock cycles  CMPCSource=Specify via dialog  CMPCValue_per=50  CMPCValue_clk=32000  enCMPCshadow=Counter equals to zero  ePWMxLINKCMPD=Not Linked  CMPDUnits=Clock cycles  CMPDSource=Specify via dialog  CMPDValue_per=50  CMPDValue_clk=32000  enCMPDshadow=Counter equals to zero  enableDBePWMxA=on  enableDBePWMxB=on  enhalfcycle=off  DBpolarity=Active high complementary (AHC)  DBedgeDelay=Positive  DBSource_ePWMxA=ePWMxA  DBSource_ePWMxB=ePWMxA  DBperiodSource=Input port  REDperiod=0  FEDperiod=0  adcstartModuleA=off  adcrequestEventA=First event  adcstartEventA=Digital Compare Module A Event 1 start of conversion (DCAEVT1.soc)  adcstartEventA_type2=Digital Compare Module A Event 1 start of conversion (DCAEVT1.soc)  adcstartModuleB=off  adcrequestEventB=First event  adcstartEventB=Counter equals to zero (CTR=Zero)  adcstartEventB_type2=Counter equals to zero (CTR=Zero)  intEn=off  intPrd=First event  intSel=Counter equals to zero (CTR=Zero)  intSel_type2=Counter equals to zero (CTR=Zero)  hrpe=off  enHRPWM=off  HRPWM_LoadMode=Counter equals to period (CTR=PRD)  HRPWM_CTLMode=Duty or Period control mode  HRPWM_EDGMode=Both edge  hrpeb=off  enHRPWMB=off  HRPWM_LoadModeB=Counter equals to zero (CTR=ZERO)  HRPWM_CTLModeB=Duty or Period control mode  HRPWM_EDGModeB=Both edge  enSFO=on  enautoconv=on  chopperEnable=off  chopperFrequency=1  chopperFirstwidth=1  chopperDuty=12.5%  tripZonesource=Specify via dialog  tzselOSHT1=off  tzselOSHT2=off  tzselOSHT3=off  tzselOSHDCAEV1=off  tzselOSHDCBEV1=off  tzselCBC1=off  tzselCBC2=off  tzselCBC3=off  tzselCBCDCAEV2=off  tzselCBCDCBEV2=off  tzselOSHT4=off  tzselOSHT5=off  tzselOSHT6=off  tzselCBC4=off  tzselCBC5=off  tzselCBC6=off  enTzOstIntr=off  enTzCbcIntr=off  enTzDCAEVT1Intr=off  enTzDCAEVT2Intr=off  enTzDCBEVT1Intr=off  enTzDCBEVT2Intr=off  ePWMxAforced=No action  ePWMxBforced=No action  DCAEVT1forced=No action  DCBEVT1forced=No action  DCAEVT2forced=No action  DCBEVT2forced=No action  dcah=Trip Zone 1 input (TZ1)  dcal=Trip Zone 2 input (TZ2)  dcbh=Trip Zone 1 input (TZ1)  dcbl=Trip Zone 2 input (TZ2)  dcah_type2=GPTRIP1SEL/(TZ1)  dcal_type2=GPTRIP2SEL/(TZ2)  dcbh_type2=GPTRIP1SEL/(TZ1)  dcbl_type2=GPTRIP2SEL/(TZ2)  gendcaevt1=Event disabled  gendcaevt2=Event disabled  gendcbevt1=Event disabled  gendcbevt2=Event disabled  dcaevt1src=DCAEVT1 with sync  dcaevt2src=DCAEVT2 with sync  dcbevt1src=DCBEVT1 with sync  dcbevt2src=DCBEVT2 with sync  pulsesel=Counter equals to zero (CTR=Zero)  blankinv=off  blankoffset=0  blankwidth=0  evsrcsel=Filtered version of DCAEVT1 (DCAEVT1FILT)  encape=off  PwmType=C2000_Type4
  ePWM1 : c2802xlib/ePWM  useModule=ePWM3  ePWMxLINKTBPRD=Not Linked  periodUnits=Clock cycles  timerSource=Specify via dialog  timerPeriod_clk=12500  timerPeriod_sec=0.0001  tbshadow=Counter equals to zero  countingMode=Up-Down  phaseActiveEnable=Disable  phaseDirection=Count down after sync  phaseActive=0  synchronizationEnable=off  dcaevt1Sync=off  dcbevt1Sync=off  synchronizationOption=Disable  clockPrescale=1  HSclockPrescale=1  enswap=off  ePWMxAStatus=on  ePWMxAactionLogic1=Set  ePWMxAactionLogic2=Clear  ePWMxAactionLogic3=Clear  ePWMxAactionLogic4=Set  ePWMxAactionLogic5=Do nothing  ePWMxAactionLogic6=Do nothing  ePWMxALoadMode=Load on counter equals to zero (CTR=Zero)  ePWMxACSFenable=off  ePWMxACSFvalue=Forcing disable  ePWMxASFreload=Zero  ePWMxBStatus=on  ePWMxBactionLogic1=Clear  ePWMxBactionLogic2=Set  ePWMxBactionLogic3=Do nothing  ePWMxBactionLogic4=Do nothing  ePWMxBactionLogic5=Set  ePWMxBactionLogic6=Clear  ePWMxBLoadMode=Load on counter equals to zero (CTR=Zero)  ePWMxBCSFenable=off  ePWMxBCSFvalue=Forcing disable  ePWMxBSFreload=Zero  ePWNxBOutWay=off  ePWMxLINKCMPA=Not Linked  CMPAUnits=Clock cycles  CMPASource=Input port  CMPAValue_per=50  CMPAValue_clk=3750  enCMPAshadow=Counter equals to zero  ePWMxLINKCMPB=Not Linked  CMPBUnits=Clock cycles  CMPBSource=Input port  CMPBValue_per=50  CMPBValue_clk=3750  enCMPBshadow=Counter equals to zero  ePWMxLINKCMPC=Not Linked  CMPCUnits=Clock cycles  CMPCSource=Specify via dialog  CMPCValue_per=50  CMPCValue_clk=32000  enCMPCshadow=Counter equals to zero  ePWMxLINKCMPD=Not Linked  CMPDUnits=Clock cycles  CMPDSource=Specify via dialog  CMPDValue_per=50  CMPDValue_clk=32000  enCMPDshadow=Counter equals to zero  enableDBePWMxA=on  enableDBePWMxB=on  enhalfcycle=off  DBpolarity=Active high complementary (AHC)  DBedgeDelay=Positive  DBSource_ePWMxA=ePWMxA  DBSource_ePWMxB=ePWMxA  DBperiodSource=Input port  REDperiod=0  FEDperiod=0  adcstartModuleA=off  adcrequestEventA=First event  adcstartEventA=Digital Compare Module A Event 1 start of conversion (DCAEVT1.soc)  adcstartEventA_type2=Digital Compare Module A Event 1 start of conversion (DCAEVT1.soc)  adcstartModuleB=off  adcrequestEventB=First event  adcstartEventB=Counter equals to zero (CTR=Zero)  adcstartEventB_type2=Counter equals to zero (CTR=Zero)  intEn=off  intPrd=First event  intSel=Counter equals to zero (CTR=Zero)  intSel_type2=Counter equals to zero (CTR=Zero)  hrpe=off  enHRPWM=off  HRPWM_LoadMode=Counter equals to period (CTR=PRD)  HRPWM_CTLMode=Duty or Period control mode  HRPWM_EDGMode=Both edge  hrpeb=off  enHRPWMB=off  HRPWM_LoadModeB=Counter equals to zero (CTR=ZERO)  HRPWM_CTLModeB=Duty or Period control mode  HRPWM_EDGModeB=Both edge  enSFO=on  enautoconv=on  chopperEnable=off  chopperFrequency=1  chopperFirstwidth=1  chopperDuty=12.5%  tripZonesource=Specify via dialog  tzselOSHT1=off  tzselOSHT2=off  tzselOSHT3=off  tzselOSHDCAEV1=off  tzselOSHDCBEV1=off  tzselCBC1=off  tzselCBC2=off  tzselCBC3=off  tzselCBCDCAEV2=off  tzselCBCDCBEV2=off  tzselOSHT4=off  tzselOSHT5=off  tzselOSHT6=off  tzselCBC4=off  tzselCBC5=off  tzselCBC6=off  enTzOstIntr=off  enTzCbcIntr=off  enTzDCAEVT1Intr=off  enTzDCAEVT2Intr=off  enTzDCBEVT1Intr=off  enTzDCBEVT2Intr=off  ePWMxAforced=No action  ePWMxBforced=No action  DCAEVT1forced=No action  DCBEVT1forced=No action  DCAEVT2forced=No action  DCBEVT2forced=No action  dcah=Trip Zone 1 input (TZ1)  dcal=Trip Zone 2 input (TZ2)  dcbh=Trip Zone 1 input (TZ1)  dcbl=Trip Zone 2 input (TZ2)  dcah_type2=GPTRIP1SEL/(TZ1)  dcal_type2=GPTRIP2SEL/(TZ2)  dcbh_type2=GPTRIP1SEL/(TZ1)  dcbl_type2=GPTRIP2SEL/(TZ2)  gendcaevt1=Event disabled  gendcaevt2=Event disabled  gendcbevt1=Event disabled  gendcbevt2=Event disabled  dcaevt1src=DCAEVT1 with sync  dcaevt2src=DCAEVT2 with sync  dcbevt1src=DCBEVT1 with sync  dcbevt2src=DCBEVT2 with sync  pulsesel=Counter equals to zero (CTR=Zero)  blankinv=off  blankoffset=0  blankwidth=0  evsrcsel=Filtered version of DCAEVT1 (DCAEVT1FILT)  encape=off  PwmType=C2000_Type4
  ePWM2 : c2802xlib/ePWM  useModule=ePWM6  ePWMxLINKTBPRD=Not Linked  periodUnits=Clock cycles  timerSource=Specify via dialog  timerPeriod_clk=12500  timerPeriod_sec=0.0001  tbshadow=Counter equals to zero  countingMode=Up-Down  phaseActiveEnable=Disable  phaseDirection=Count down after sync  phaseActive=0  synchronizationEnable=off  dcaevt1Sync=off  dcbevt1Sync=off  synchronizationOption=Disable  clockPrescale=1  HSclockPrescale=1  enswap=off  ePWMxAStatus=on  ePWMxAactionLogic1=Set  ePWMxAactionLogic2=Clear  ePWMxAactionLogic3=Clear  ePWMxAactionLogic4=Set  ePWMxAactionLogic5=Do nothing  ePWMxAactionLogic6=Do nothing  ePWMxALoadMode=Load on counter equals to zero (CTR=Zero)  ePWMxACSFenable=off  ePWMxACSFvalue=Forcing disable  ePWMxASFreload=Zero  ePWMxBStatus=on  ePWMxBactionLogic1=Clear  ePWMxBactionLogic2=Set  ePWMxBactionLogic3=Do nothing  ePWMxBactionLogic4=Do nothing  ePWMxBactionLogic5=Set  ePWMxBactionLogic6=Clear  ePWMxBLoadMode=Load on counter equals to zero (CTR=Zero)  ePWMxBCSFenable=off  ePWMxBCSFvalue=Forcing disable  ePWMxBSFreload=Zero  ePWNxBOutWay=off  ePWMxLINKCMPA=Not Linked  CMPAUnits=Clock cycles  CMPASource=Input port  CMPAValue_per=50  CMPAValue_clk=3750  enCMPAshadow=Counter equals to zero  ePWMxLINKCMPB=Not Linked  CMPBUnits=Clock cycles  CMPBSource=Input port  CMPBValue_per=50  CMPBValue_clk=3750  enCMPBshadow=Counter equals to zero  ePWMxLINKCMPC=Not Linked  CMPCUnits=Clock cycles  CMPCSource=Specify via dialog  CMPCValue_per=50  CMPCValue_clk=32000  enCMPCshadow=Counter equals to zero  ePWMxLINKCMPD=Not Linked  CMPDUnits=Clock cycles  CMPDSource=Specify via dialog  CMPDValue_per=50  CMPDValue_clk=32000  enCMPDshadow=Counter equals to zero  enableDBePWMxA=on  enableDBePWMxB=on  enhalfcycle=off  DBpolarity=Active high complementary (AHC)  DBedgeDelay=Positive  DBSource_ePWMxA=ePWMxA  DBSource_ePWMxB=ePWMxA  DBperiodSource=Input port  REDperiod=0  FEDperiod=0  adcstartModuleA=off  adcrequestEventA=First event  adcstartEventA=Digital Compare Module A Event 1 start of conversion (DCAEVT1.soc)  adcstartEventA_type2=Digital Compare Module A Event 1 start of conversion (DCAEVT1.soc)  adcstartModuleB=off  adcrequestEventB=First event  adcstartEventB=Counter equals to zero (CTR=Zero)  adcstartEventB_type2=Counter equals to zero (CTR=Zero)  intEn=off  intPrd=First event  intSel=Counter equals to zero (CTR=Zero)  intSel_type2=Counter equals to zero (CTR=Zero)  hrpe=off  enHRPWM=off  HRPWM_LoadMode=Counter equals to period (CTR=PRD)  HRPWM_CTLMode=Duty or Period control mode  HRPWM_EDGMode=Both edge  hrpeb=off  enHRPWMB=off  HRPWM_LoadModeB=Counter equals to zero (CTR=ZERO)  HRPWM_CTLModeB=Duty or Period control mode  HRPWM_EDGModeB=Both edge  enSFO=on  enautoconv=on  chopperEnable=off  chopperFrequency=1  chopperFirstwidth=1  chopperDuty=12.5%  tripZonesource=Specify via dialog  tzselOSHT1=off  tzselOSHT2=off  tzselOSHT3=off  tzselOSHDCAEV1=off  tzselOSHDCBEV1=off  tzselCBC1=off  tzselCBC2=off  tzselCBC3=off  tzselCBCDCAEV2=off  tzselCBCDCBEV2=off  tzselOSHT4=off  tzselOSHT5=off  tzselOSHT6=off  tzselCBC4=off  tzselCBC5=off  tzselCBC6=off  enTzOstIntr=off  enTzCbcIntr=off  enTzDCAEVT1Intr=off  enTzDCAEVT2Intr=off  enTzDCBEVT1Intr=off  enTzDCBEVT2Intr=off  ePWMxAforced=No action  ePWMxBforced=No action  DCAEVT1forced=No action  DCBEVT1forced=No action  DCAEVT2forced=No action  DCBEVT2forced=No action  dcah=Trip Zone 1 input (TZ1)  dcal=Trip Zone 2 input (TZ2)  dcbh=Trip Zone 1 input (TZ1)  dcbl=Trip Zone 2 input (TZ2)  dcah_type2=GPTRIP1SEL/(TZ1)  dcal_type2=GPTRIP2SEL/(TZ2)  dcbh_type2=GPTRIP1SEL/(TZ1)  dcbl_type2=GPTRIP2SEL/(TZ2)  gendcaevt1=Event disabled  gendcaevt2=Event disabled  gendcbevt1=Event disabled  gendcbevt2=Event disabled  dcaevt1src=DCAEVT1 with sync  dcaevt2src=DCAEVT2 with sync  dcbevt1src=DCBEVT1 with sync  dcbevt2src=DCBEVT2 with sync  pulsesel=Counter equals to zero (CTR=Zero)  blankinv=off  blankoffset=0  blankwidth=0  evsrcsel=Filtered version of DCAEVT1 (DCAEVT1FILT)  encape=off  PwmType=C2000_Type4
  ePWM3 : c2802xlib/ePWM  useModule=ePWM4  ePWMxLINKTBPRD=Not Linked  periodUnits=Clock cycles  timerSource=Specify via dialog  timerPeriod_clk=12500  timerPeriod_sec=0.0001  tbshadow=Counter equals to zero  countingMode=Up-Down  phaseActiveEnable=Disable  phaseDirection=Count down after sync  phaseActive=0  synchronizationEnable=off  dcaevt1Sync=off  dcbevt1Sync=off  synchronizationOption=Disable  clockPrescale=1  HSclockPrescale=1  enswap=off  ePWMxAStatus=on  ePWMxAactionLogic1=Set  ePWMxAactionLogic2=Clear  ePWMxAactionLogic3=Clear  ePWMxAactionLogic4=Set  ePWMxAactionLogic5=Do nothing  ePWMxAactionLogic6=Do nothing  ePWMxALoadMode=Load on counter equals to zero (CTR=Zero)  ePWMxACSFenable=off  ePWMxACSFvalue=Forcing disable  ePWMxASFreload=Zero  ePWMxBStatus=on  ePWMxBactionLogic1=Clear  ePWMxBactionLogic2=Set  ePWMxBactionLogic3=Do nothing  ePWMxBactionLogic4=Do nothing  ePWMxBactionLogic5=Set  ePWMxBactionLogic6=Clear  ePWMxBLoadMode=Load on counter equals to zero (CTR=Zero)  ePWMxBCSFenable=off  ePWMxBCSFvalue=Forcing disable  ePWMxBSFreload=Zero  ePWNxBOutWay=off  ePWMxLINKCMPA=Not Linked  CMPAUnits=Clock cycles  CMPASource=Input port  CMPAValue_per=50  CMPAValue_clk=3750  enCMPAshadow=Counter equals to zero  ePWMxLINKCMPB=Not Linked  CMPBUnits=Clock cycles  CMPBSource=Input port  CMPBValue_per=50  CMPBValue_clk=3750  enCMPBshadow=Counter equals to zero  ePWMxLINKCMPC=Not Linked  CMPCUnits=Clock cycles  CMPCSource=Specify via dialog  CMPCValue_per=50  CMPCValue_clk=32000  enCMPCshadow=Counter equals to zero  ePWMxLINKCMPD=Not Linked  CMPDUnits=Clock cycles  CMPDSource=Specify via dialog  CMPDValue_per=50  CMPDValue_clk=32000  enCMPDshadow=Counter equals to zero  enableDBePWMxA=on  enableDBePWMxB=on  enhalfcycle=off  DBpolarity=Active high complementary (AHC)  DBedgeDelay=Positive  DBSource_ePWMxA=ePWMxA  DBSource_ePWMxB=ePWMxA  DBperiodSource=Input port  REDperiod=0  FEDperiod=0  adcstartModuleA=off  adcrequestEventA=First event  adcstartEventA=Digital Compare Module A Event 1 start of conversion (DCAEVT1.soc)  adcstartEventA_type2=Digital Compare Module A Event 1 start of conversion (DCAEVT1.soc)  adcstartModuleB=off  adcrequestEventB=First event  adcstartEventB=Counter equals to zero (CTR=Zero)  adcstartEventB_type2=Counter equals to zero (CTR=Zero)  intEn=off  intPrd=First event  intSel=Counter equals to zero (CTR=Zero)  intSel_type2=Counter equals to zero (CTR=Zero)  hrpe=off  enHRPWM=off  HRPWM_LoadMode=Counter equals to period (CTR=PRD)  HRPWM_CTLMode=Duty or Period control mode  HRPWM_EDGMode=Both edge  hrpeb=off  enHRPWMB=off  HRPWM_LoadModeB=Counter equals to zero (CTR=ZERO)  HRPWM_CTLModeB=Duty or Period control mode  HRPWM_EDGModeB=Both edge  enSFO=on  enautoconv=on  chopperEnable=off  chopperFrequency=1  chopperFirstwidth=1  chopperDuty=12.5%  tripZonesource=Specify via dialog  tzselOSHT1=off  tzselOSHT2=off  tzselOSHT3=off  tzselOSHDCAEV1=off  tzselOSHDCBEV1=off  tzselCBC1=off  tzselCBC2=off  tzselCBC3=off  tzselCBCDCAEV2=off  tzselCBCDCBEV2=off  tzselOSHT4=off  tzselOSHT5=off  tzselOSHT6=off  tzselCBC4=off  tzselCBC5=off  tzselCBC6=off  enTzOstIntr=off  enTzCbcIntr=off  enTzDCAEVT1Intr=off  enTzDCAEVT2Intr=off  enTzDCBEVT1Intr=off  enTzDCBEVT2Intr=off  ePWMxAforced=No action  ePWMxBforced=No action  DCAEVT1forced=No action  DCBEVT1forced=No action  DCAEVT2forced=No action  DCBEVT2forced=No action  dcah=Trip Zone 1 input (TZ1)  dcal=Trip Zone 2 input (TZ2)  dcbh=Trip Zone 1 input (TZ1)  dcbl=Trip Zone 2 input (TZ2)  dcah_type2=GPTRIP1SEL/(TZ1)  dcal_type2=GPTRIP2SEL/(TZ2)  dcbh_type2=GPTRIP1SEL/(TZ1)  dcbl_type2=GPTRIP2SEL/(TZ2)  gendcaevt1=Event disabled  gendcaevt2=Event disabled  gendcbevt1=Event disabled  gendcbevt2=Event disabled  dcaevt1src=DCAEVT1 with sync  dcaevt2src=DCAEVT2 with sync  dcbevt1src=DCBEVT1 with sync  dcbevt2src=DCBEVT2 with sync  pulsesel=Counter equals to zero (CTR=Zero)  blankinv=off  blankoffset=0  blankwidth=0  evsrcsel=Filtered version of DCAEVT1 (DCAEVT1FILT)  encape=off  PwmType=C2000_Type4
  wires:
  PWM/1 -> Demux5/1
  Product/1 -> Product15/1
  Add/1 -> Product/1
  Add14/1 -> Product18/1
  Add13/1 -> Product16/1
  Product18/1 -> Product19/1
  Product16/1 -> Product17/1
  Constant15/1 -> Add15/2, Add/2, Add13/2, Add14/2
  Product20/1 -> Product21/1
  Add15/1 -> Product20/1
  Constant14/1 -> Product17/2, Product21/2, Product15/2, Product19/2
  Constant13/1 -> Product18/2, Product16/2, Product20/2, Product/2
  Demux5/1 -> Add15/1
  Demux5/2 -> Add/1
  Demux5/3 -> Add13/1
  Demux5/4 -> Add14/1
  Product19/1 -> ePWM3/1, ePWM3/2
  Product15/1 -> ePWM2/1, ePWM2/2
  Product17/1 -> ePWM1/1, ePWM1/2
  Product21/1 -> ePWM/1, ePWM/2
  DeadBand/1 -> ePWM/4, ePWM2/4, ePWM3/4, ePWM1/4, ePWM/3, ePWM2/3, ePWM3/3, ePWM1/3

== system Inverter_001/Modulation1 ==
  Vcontrol : Inport
  VDC : Inport  Port=2
  Add16 : Sum
  Add17 : Sum
  Add18 : Sum
  Carrier1 : Subsystem
  Demux4 : Demux  Outputs=3
  Float to IQN1 : tiiqmathlib/Float to IQN  Q_value=10
  Gain : Gain  Gain=0.5  OutDataTypeStr=single
  IQN / IQN : tiiqmathlib/IQN // IQN
  IQN / IQN1 : tiiqmathlib/IQN // IQN
  IQN / IQN2 : tiiqmathlib/IQN // IQN
  Mux6 : Mux
  Mux7 : Mux  Inputs=3
  VPWM : Outport
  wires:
  Add17/1 -> Mux6/2  "PhaseB"
  Carrier1/1(Out1) -> Mux6/4, Add16/2, Add17/2, Add18/2  "PhaseN"
  Demux4/2 -> IQN / IQN1/1
  Add16/1 -> Mux6/1  "PhaseA"
  Mux7/1 -> Carrier1/1(In1)
  IQN / IQN1/1 -> Mux7/2, Add17/1
  Demux4/1 -> IQN / IQN/1
  Mux6/1 -> VPWM/1
  Demux4/3 -> IQN / IQN2/1
  VDC/1 -> Gain/1
  Add18/1 -> Mux6/3  "PhaseC"
  IQN / IQN2/1 -> Mux7/3, Add18/1
  Gain/1 -> Float to IQN1/1
  Vcontrol/1 -> Demux4/1
  Float to IQN1/1 -> IQN / IQN1/2, IQN / IQN/2, IQN / IQN2/2
  IQN / IQN/1 -> Mux7/1, Add16/1

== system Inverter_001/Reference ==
  note: Red: Set Sample Time
  Vac Ref : Inport
  Constant10 : Constant  Value=0  OutDataTypeStr=single
  Constant11 : Constant  Value=0.005  OutDataTypeStr=fixdt(1,32,2^-29,0)
  Constant13 : Constant  OutDataTypeStr=single
  Constant14 : Constant  Value=0  OutDataTypeStr=single
  Constant8 : Constant  OutDataTypeStr=fixdt(1,32,2^-29,0)  SampleTime=-1
  Constant9 : Constant  Value=0  OutDataTypeStr=fixdt(1,32,2^-29,0)
  Float to IQN : tiiqmathlib/Float to IQN  Q_value=10
  Float to IQN1 : tiiqmathlib/Float to IQN  Q_value=10
  Float to IQN2 : tiiqmathlib/Float to IQN  Q_value=10
  Gain2 : Gain  Gain=2*pi
  Gain3 : Gain  Gain=sqrt(2)  OutDataTypeStr=Inherit: Inherit via back propagation
  IQN to Float3 : tiiqmathlib/IQN to Float
  Inverse Park Transformation : Subsystem  InitFcn=tic2000lib_licenseCheck  mask(Inverse Park Transformation){}
      mask help: This block performs vector transformation from orthogonal rotating reference frame into orthogonal stationary frame. All inputs and outputs are signed 32-bit fixed-point numbers with Q value between 1 and 29.
  Mux2 : Mux  Inputs=3
  Product5 : Product
  Ramp Generator1 : c28xdmclib/Ramp Generator  step_angle_max=1
  abc : Outport
  angle : Outport  Port=2
  dq0 : Outport  Port=3
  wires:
  Vac Ref/1 -> Gain3/1
  IQN to Float3/1 -> Gain2/1
  Constant11/1 -> Ramp Generator1/3
  Gain2/1 -> Float to IQN1/1
  Constant14/1 -> Mux2/2
  Constant9/1 -> Ramp Generator1/2
  Float to IQN2/1 -> Product5/2
  Constant10/1 -> Mux2/3
  Product5/1 -> Float to IQN/1
  Constant13/1 -> Mux2/1
  Mux2/1 -> Product5/1
  Float to IQN1/1 -> angle/1, Inverse Park Transformation/2(theta)
  Constant8/1 -> Ramp Generator1/1
  Float to IQN/1 -> dq0/1, Inverse Park Transformation/1(DQ0)
  Gain3/1 -> Float to IQN2/1
  Ramp Generator1/1 -> IQN to Float3/1
  Inverse Park Transformation/1(ABC) -> abc/1

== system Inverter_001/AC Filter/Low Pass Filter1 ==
  Input : Inport
  TimeConstant : Inport  Port=2
  IQN1 x IQN2 : tiiqmathlib/IQN1 x IQN2  Q=10
  Sum1 : Sum  Inputs=|+-  AccumDataTypeStr=single
  Sum2 : Sum  Inputs=|++  AccumDataTypeStr=single
  Sum3 : Sum  Inputs=|+-
  Unit Delay : UnitDelay  SampleTime=-1
  Unit Delay1 : UnitDelay  SampleTime=-1
  Output : Outport
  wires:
  Sum3/1 -> Output/1  "HighPassFilterOutput"
  Unit Delay1/1 -> Sum2/2
  TimeConstant/1 -> IQN1 x IQN2/1  "tc"
  Unit Delay/1 -> Sum2/1
  Sum2/1 -> IQN1 x IQN2/2, Unit Delay1/1  "state"
  Sum1/1 -> Unit Delay/1, Sum3/2  "HighPassFilterOutput"
  IQN1 x IQN2/1 -> Sum1/2  "TcState"
  Input/1 -> Sum1/1, Sum3/1
